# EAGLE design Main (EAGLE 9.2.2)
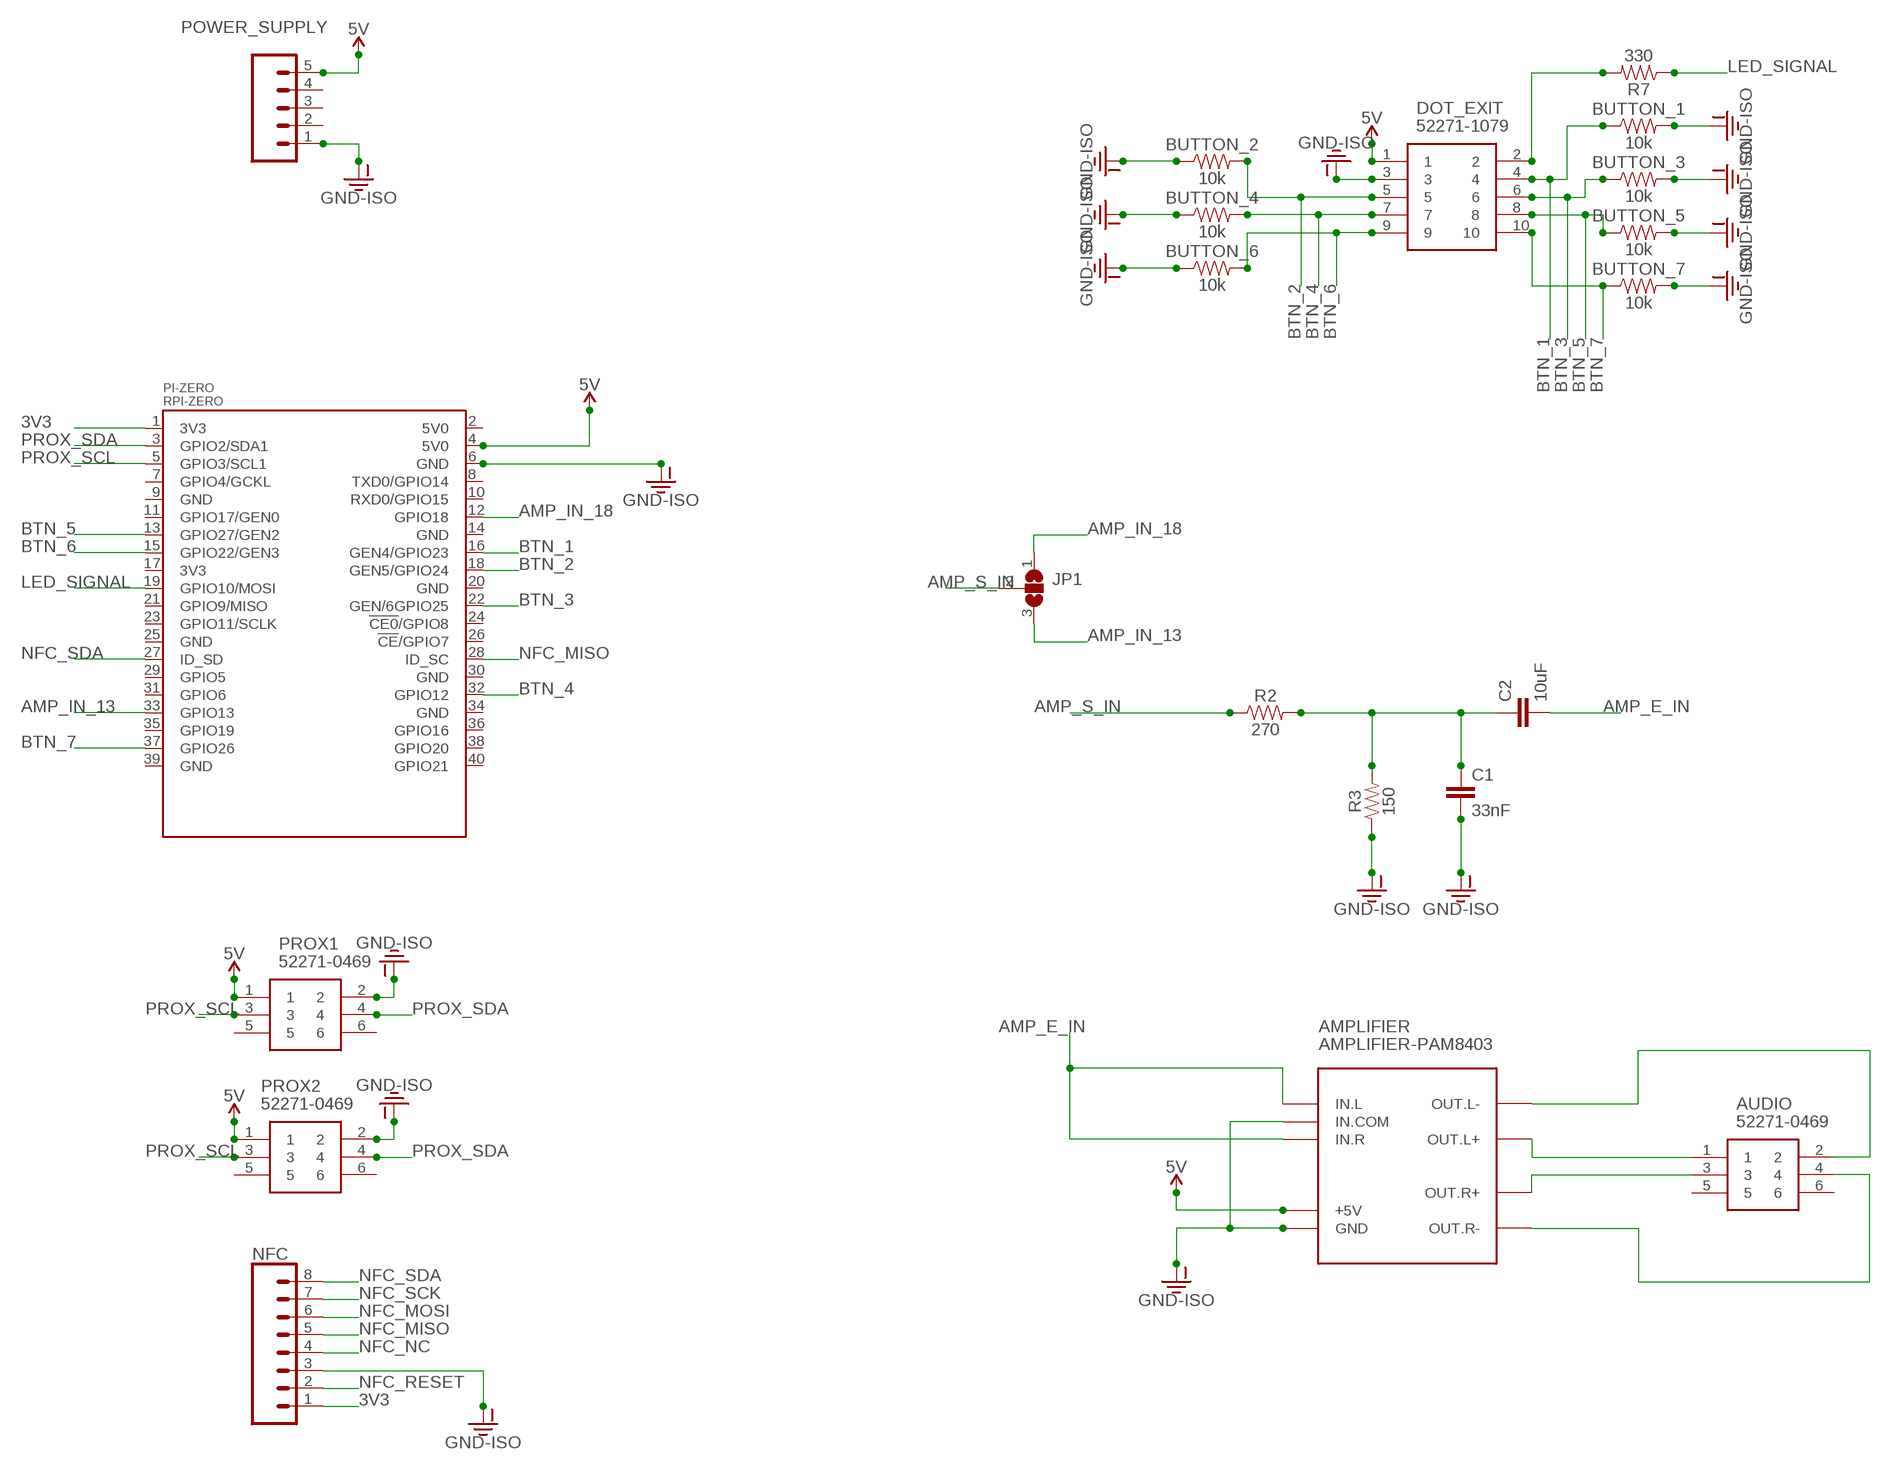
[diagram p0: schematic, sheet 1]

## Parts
AMPLIFIER  AMPLIFIER-PAM8403  [AMPLIFIER-PAM8403]
AUDIO  52271-0469  [MOLEX_52271-0469]
BUTTON_1  10k  1KOHM-HORIZ-1/4W-1%  [AXIAL-0.3]
BUTTON_2  10k  1KOHM-HORIZ-1/4W-1%  [AXIAL-0.3]
BUTTON_3  10k  1KOHM-HORIZ-1/4W-1%  [AXIAL-0.3]
BUTTON_4  10k  1KOHM-HORIZ-1/4W-1%  [AXIAL-0.3]
BUTTON_5  10k  1KOHM-HORIZ-1/4W-1%  [AXIAL-0.3]
BUTTON_6  10k  1KOHM-HORIZ-1/4W-1%  [AXIAL-0.3]
BUTTON_7  10k  1KOHM-HORIZ-1/4W-1%  [AXIAL-0.3]
C1  33nF  10NF-PTH-10MM-10000V-1-%  [CAP-PTH-10MM]
C2  10uF  10NF-PTH-10MM-10000V-1-%  [CAP-PTH-10MM]
DOT_EXIT  52271-1079  [52271-1079]
JP1  SJ2W  [SJ_2]
NFC  CONN_08"  [1X08]
PI-ZERO  RPI-ZERO  [RASPBERRYPI_BASTELSTUBE_V13_RASPI_BOARD_B+_FULL]
POWER_SUPPLY  CONN_05  [1X05]
PROX1  52271-0469  [MOLEX_52271-0469]
PROX2  52271-0469  [MOLEX_52271-0469]
R2  270  330OHM-HORIZ-1/10W-5%  [AXIAL-0.3]
R3  150  330OHM-HORIZ-1/10W-5%  [AXIAL-0.3]
R7  330  330OHM-HORIZ-1/10W-5%  [AXIAL-0.3]

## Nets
3V3: NFC.1 PI-ZERO.1(3V3)
5V [power]: AMPLIFIER.+5V DOT_EXIT.1 PI-ZERO.4(5V0) POWER_SUPPLY.5 PROX1.1 PROX2.1
AMP_E_IN: AMPLIFIER.IN.L AMPLIFIER.IN.R C2.2
AMP_IN_13: JP1.3 PI-ZERO.33(GPIO13)
AMP_IN_18: JP1.1 PI-ZERO.12(GPIO18)
AMP_S_IN: JP1.2 R2.P$1
BTN_1: BUTTON_1.P$1 DOT_EXIT.4 PI-ZERO.16(GEN4/GPIO23)
BTN_2: BUTTON_2.P$2 DOT_EXIT.5 PI-ZERO.18(GEN5/GPIO24)
BTN_3: BUTTON_3.P$1 DOT_EXIT.6 PI-ZERO.22(GEN/6GPIO25)
BTN_4: BUTTON_4.P$2 DOT_EXIT.7 PI-ZERO.32(GPIO12)
BTN_5: BUTTON_5.P$1 DOT_EXIT.8 PI-ZERO.13(GPIO27/GEN2)
BTN_6: BUTTON_6.P$2 DOT_EXIT.9 PI-ZERO.15(GPIO22/GEN3)
BTN_7: BUTTON_7.P$1 DOT_EXIT.10 PI-ZERO.37(GPIO26)
GND-ISO [power]: AMPLIFIER.GND AMPLIFIER.IN.COM BUTTON_1.P$2 BUTTON_2.P$1 BUTTON_3.P$2 BUTTON_4.P$1 BUTTON_5.P$2 BUTTON_6.P$1 BUTTON_7.P$2 C1.2 DOT_EXIT.3 NFC.3 PI-ZERO.6(GND) POWER_SUPPLY.1 PROX1.2 PROX2.2 R3.P$1
LED_SIGNAL: PI-ZERO.19(GPIO10/MOSI) R7.P$1
N$1: DOT_EXIT.2 R7.P$2
N$2: AMPLIFIER.OUT.L- AUDIO.2
N$3: AMPLIFIER.OUT.L+ AUDIO.1
N$4: C1.1 C2.1 R2.P$2 R3.P$2
N$5: AMPLIFIER.OUT.R+ AUDIO.3
N$6: AMPLIFIER.OUT.R- AUDIO.4
NFC_MISO: NFC.5 PI-ZERO.28(ID_SC)
NFC_MOSI: NFC.6
NFC_NC: NFC.4
NFC_RESET: NFC.2
NFC_SCK: NFC.7
NFC_SDA: NFC.8 PI-ZERO.27(ID_SD)
PROX_SCL: PI-ZERO.5(GPIO3/SCL1) PROX1.3 PROX2.3
PROX_SDA: PI-ZERO.3(GPIO2/SDA1) PROX1.4 PROX2.4
Unconnected: AUDIO.5 AUDIO.6 PI-ZERO.2(5V0) PI-ZERO.7(GPIO4/GCKL) PI-ZERO.8(TXD0/GPIO14) PI-ZERO.9(GND) PI-ZERO.10(RXD0/GPIO15) PI-ZERO.11(GPIO17/GEN0) PI-ZERO.14(GND) PI-ZERO.17(3V3) PI-ZERO.20(GND) PI-ZERO.21(GPIO9/MISO) PI-ZERO.23(GPIO11/SCLK) PI-ZERO.24(!CE0!/GPIO8) PI-ZERO.25(GND) PI-ZERO.26(!CE!/GPIO7) PI-ZERO.29(GPIO5) PI-ZERO.30(GND) PI-ZERO.31(GPIO6) PI-ZERO.34(GND) PI-ZERO.35(GPIO19) PI-ZERO.36(GPIO16) PI-ZERO.38(GPIO20) PI-ZERO.39(GND) PI-ZERO.40(GPIO21) POWER_SUPPLY.2 POWER_SUPPLY.3 POWER_SUPPLY.4 PROX1.5 PROX1.6 PROX2.5 PROX2.6

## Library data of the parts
AMPLIFIER = diy-modules:AMPLIFIER-PAM8403: Stereo Class-D 3W Audio Amplifier based on PAM8403 chip More details available here: http://artofcircuits.com/product/pam8403-5v-two-channel-stereo-mini-class-d-3w3w-audio-amplifier Click here to find device on ebay.com
AUDIO PROX1 PROX2 = 52271-0469:52271-0469: CONNECTOR, FPC, 1.0MM, 4 WAY Source: Datasheet; ALLIED_NUMBER: 70374312; DESCRIPTION: CONNECTOR, FPC, 1.0MM, 4 WAY; HEIGHT: mm; MANUFACTURER_NAME: Molex; MANUFACTURER_PART_NUMBER: 52271-0469; RS_PART_NUMBER: 1707199
BUTTON_1-BUTTON_7 = SparkFun-Resistors:1KOHM: 1kΩ resistor; PROD_ID: RES-12182; VALUE: 1k
C1 C2 = SparkFun-Capacitors:10NF: 0.01uF/10nF/10,000pF ceramic capacitors; PROD_ID: CAP-09321; VALUE: 10nF
DOT_EXIT = 52271-1079:52271-1079: 1.0MM FPC R/A CONN 10 W Molex FFC/FPC SMT Series 1mm Pitch 10 Way Right Angle SMT Female FPC Connector, ZIF Bottom Contact Source: Datasheet; ALLIED_NUMBER: 70373119; DESCRIPTION: 1.0MM FPC R/A CONN 10 W Molex FFC/FPC SMT Series 1mm Pitch 10 Way Right Angle SMT Female FPC Connector, ZIF Bottom Contact; HEIGHT: mm; MANUFACTURER_NAME: Molex; MANUFACTURER_PART_NUMBER: 52271-1079; RS_PART_NUMBER: 5144329P
JP1 = jumper:SJ2W: SMD solder JUMPER
NFC = SparkFun-Connectors:CONN_08: Multi connection point. Often used as Generic Header-pin footprint for 0.1 inch spaced/style header connections On any of the 0.1 inch spaced packages, you can populate with these: Break Away Headers - Straight (PRT-00116) Break Away Male Headers - Right Angle (PRT-00553) Female Headers (PRT-00115)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; PROD_ID: CONN-08438
PI-ZERO = RPI-Zero-Footprint:RPI-ZERO
POWER_SUPPLY = SparkFun-Connectors:CONN_05: Multi connection point. Often used as Generic Header-pin footprint for 0.1 inch spaced/style header connections On any of the 0.1 inch spaced packages, you can populate with these: Break Away Headers - Straight (PRT-00116) Break Away Male Headers - Right Angle (PRT-00553) Female Headers (PRT-00115)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
R2 R3 = SparkFun-Resistors:330OHM: 330Ω resistor; PROD_ID: RES-8371; VALUE: 330
R7 = SparkFun-Resistors:330OHM: 330Ω resistor; PROD_ID: RES-8371

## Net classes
0 default: width 0.254 mm, drill 0.508 mm, clearance 0.254 mm
1 power: width 0.508 mm, drill 0.635 mm, clearance 0.381 mm

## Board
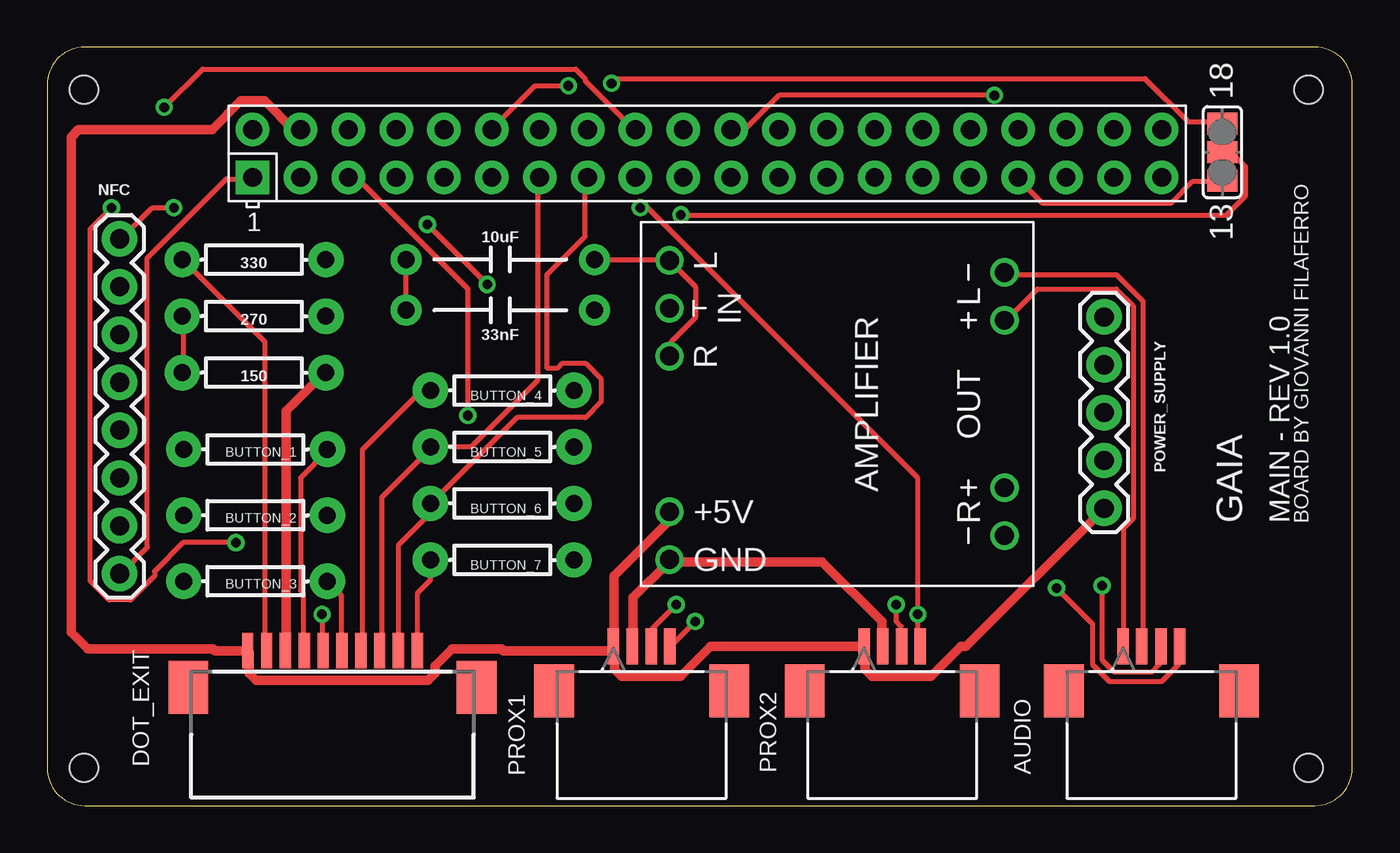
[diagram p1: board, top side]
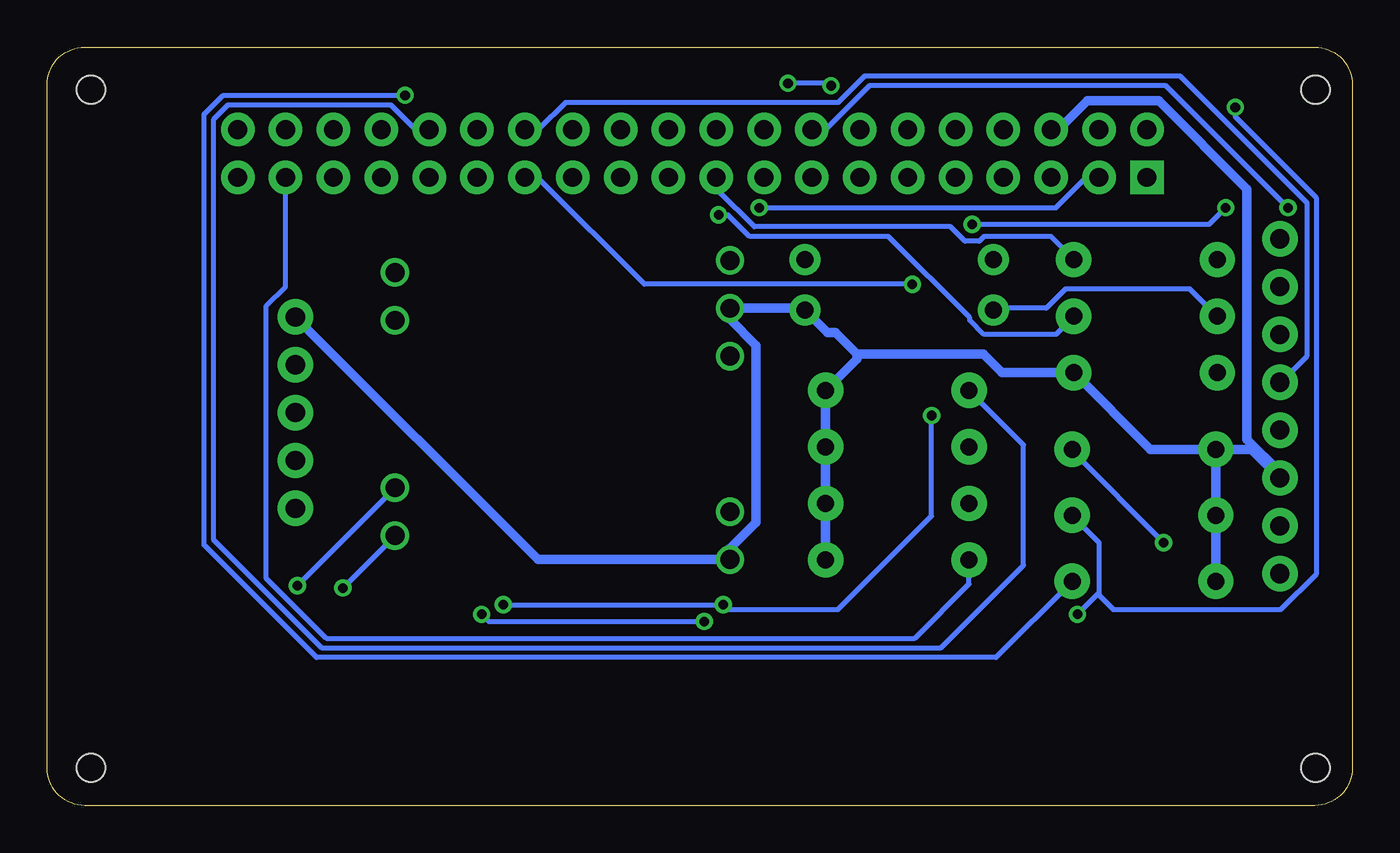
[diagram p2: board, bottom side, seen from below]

Size 69.29 x 40.27 mm. Coordinates in mm from the lower left corner, seen from the top.
Outline: 0,38.27 0,2 arc90 2,0 67.29,0 arc90 69.29,2 69.29,38.27 arc90 67.29,40.27 2,40.27 arc90 0,38.27
Copper layers (1*16): Top 0.035mm / dielectric 1.5mm / Bottom 0.035mm
Design rules "default": minimum track width 6mil, minimum drill 0.35mm, track to track 6mil, track to pad 6mil, pad to pad 6mil, via to via 6mil, smd to smd 6mil, copper to edge 40mil, drill to drill 6mil, minimum pad ring 10mil, minimum via ring 8mil, stop-mask expansion 4mil, vias tented up to drill 0mil, thermal gap 10mil
Holes 1.5 mm at 1.96,38 66.96,38 66.96,2 1.96,2

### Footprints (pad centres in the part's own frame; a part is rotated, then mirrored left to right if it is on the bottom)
AMPLIFIER-PAM8403 = drill 1: +5V 5.715,-8.89; GND 8.255,-8.89; IN.COM -5.08,-8.89; IN.L -7.62,-8.89; IN.R -2.54,-8.89; OUT.L+ -4.445,8.89; OUT.L- -6.985,8.89; OUT.R+ 4.445,8.89; OUT.R- 6.985,8.89
MOLEX_52271-0469 = smd 0.61 x 1.905: 1 1.499,4.699; 2 0.508,4.699; 3 -0.508,4.699; 4 -1.499,4.699 | smd 2.108 x 2.794: 5 -4.648,7.061; 6 4.648,7.061
AXIAL-0.3 = drill 0.9 pad 1.88: P$1 -3.81,0; P$2 3.81,0
CAP-PTH-10MM = drill 0.9 pad 1.651: 1 -5,0; 2 5,0
52271-1079 = smd 0.6 x 1.9: 1 -4.5,1.1; 2 -3.5,1.1; 3 -2.5,1.1; 4 -1.5,1.1; 5 -0.5,1.1; 6 0.5,1.1; 7 1.5,1.1; 8 2.5,1.1; 9 3.5,1.1; 10 4.5,1.1 | smd 2.1 x 2.8: 11 7.65,-0.85; 12 -7.65,-0.85
SJ_2 = smd 1.168 x 1.6: 1 -1.524,0; 2 0,0; 3 1.524,0
1X08 = drill 1.016 pad 1.88: 1 0,0; 2 2.54,0; 3 5.08,0; 4 7.62,0; 5 10.16,0; 6 12.7,0; 7 15.24,0; 8 17.78,0
RASPBERRYPI_BASTELSTUBE_V13_RASPI_BOARD_B+_FULL = drill 1 pad 1.778 square: 1 8.37,25.23 | drill 1 pad 1.778: 2 8.37,27.77; 3 10.91,25.23; 4 10.91,27.77; 5 13.45,25.23; 6 13.45,27.77; 7 15.99,25.23; 8 15.99,27.77; 9 18.53,25.23; 10 18.53,27.77; 11 21.07,25.23; 12 21.07,27.77; 13 23.61,25.23; 14 23.61,27.77; 15 26.15,25.23; 16 26.15,27.77; 17 28.69,25.23; 18 28.69,27.77; 19 31.23,25.23; 20 31.23,27.77; 21 33.77,25.23; 22 33.77,27.77; 23 36.31,25.23; 24 36.31,27.77; 25 38.85,25.23; 26 38.85,27.77; 27 41.39,25.23; 28 41.39,27.77; 29 43.93,25.23; 30 43.93,27.77; 31 46.47,25.23; 32 46.47,27.77; 33 49.01,25.23; 34 49.01,27.77; 35 51.55,25.23; 36 51.55,27.77; 37 54.09,25.23; 38 54.09,27.77; 39 56.63,25.23; 40 56.63,27.77
1X05 = drill 1.016 pad 1.88: 1 0,0; 2 2.54,0; 3 5.08,0; 4 7.62,0; 5 10.16,0

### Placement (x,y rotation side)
AMPLIFIER  41.93,21.32 270 top
AUDIO  58.62,13.15 180 top
BUTTON_1  11.06,18.91 180 top
BUTTON_2  11.06,15.41 0 top
BUTTON_3  11.06,11.91 180 top
BUTTON_4  24.16,22.04 180 top
BUTTON_5  24.16,19.04 0 top
BUTTON_6  24.16,16.04 180 top
BUTTON_7  24.16,13.04 0 top
C1  24.05,26.3 0 top
C2  24.05,28.99 0 top
DOT_EXIT  15.15,7.12 0 top
JP1  62.38,34.69 270 top
NFC  3.85,12.31 90 top
PI-ZERO  2.54,8.12 0 top
POWER_SUPPLY  56.11,25.94 270 top
PROX1  31.56,13.15 180 top
PROX2  44.86,13.15 180 top
R2  10.98,25.98 180 top
R3  10.98,22.98 180 top
R7  10.98,28.98 180 top

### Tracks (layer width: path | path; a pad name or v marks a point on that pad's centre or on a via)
3V3
  Top 0.254: PI-ZERO.1 10.79,33.27 9.52,33.27 5.33,29.07 5.33,13.71 3.93,12.31 NFC.1
5V
  Top 0.508: POWER_SUPPLY.5 48.78,8.45 48.51,8.45 46.93,6.86 43.78,6.86 43.41,7.23 43.41,8.4 PROX2.1 35.21,8.45 33.63,6.86 30.48,6.86 30.11,7.23 30.11,8.4 PROX1.1 | PROX1.1 29.83,8.22 24.2,8.22 24.11,8.3 21.49,8.3 20.59,7.4 20.59,7.01 20.21,6.63 11.09,6.63 10.71,7.01 10.71,8.16 DOT_EXIT.1 8.9,8.22 8.81,8.3 2.16,8.3 1.27,9.19 1.27,35.5 1.66,35.89 8.75,35.89 10.28,37.41 11.54,37.41 13.07,35.89 PI-ZERO.4 | AMPLIFIER.+5V 33.01,15.49 33.01,15.11 30.09,12.18 30.09,8.63 PROX1.1
AMP_E_IN
  Top 0.254: AMPLIFIER.IN.R 33.14,23.87 33.14,24.63 34.41,25.9 34.41,27.55 33.14,28.82 AMPLIFIER.IN.L 33.01,28.95 29.07,28.95 C2.2
AMP_IN_13
  Top 0.254: JP1.3 62.35,33.14 60.83,33.14 59.68,32 52.82,32 51.55,33.27 PI-ZERO.33
AMP_IN_18  (via drill 0.51)
  Top 0.254: v29.96,38.35 30.22,38.6 58.29,38.6 60.57,36.31 62.35,36.31 JP1.1 | v27.68,38.22 25.9,38.22 23.61,35.93 PI-ZERO.12
  Bottom 0.254: v29.96,38.35 27.8,38.35 v27.68,38.22
AMP_S_IN  (via drill 0.51)
  Top 0.254: v33.65,31.36 62.6,31.36 63.62,32.38 63.62,33.9 62.86,34.66 62.48,34.66 JP1.2
  Bottom 0.254: v33.65,31.36 33.14,31.36 32,30.22 24.63,30.22 20.31,25.9 20.31,25.77 19.55,25.01 15.74,25.01 14.85,25.9 R2.P$1
BTN_1  (via drill 0.51)
  Top 0.254: DOT_EXIT.4 13.58,8.25 13.58,11.29 13.45,11.42 13.45,17.39 14.85,18.79 BUTTON_1.P$1 | v3.42,31.74 2.28,30.6 2.28,11.93 3.29,10.91 4.44,10.91 5.71,12.18 5.71,12.44 7.23,13.96 v10.02,13.96
  Bottom 0.254: v3.42,31.74 9.9,38.22 25.65,38.22 27.93,35.93 28.57,35.93 PI-ZERO.16 | v10.02,13.96 14.85,18.79 BUTTON_1.P$1
BTN_2  (via drill 0.51)
  Top 0.254: v14.6,10.15 14.6,8.25 DOT_EXIT.5 | v6.22,37.08 8.25,39.11 28.06,39.11 28.57,38.6 28.57,38.47 31.11,35.93 PI-ZERO.18
  Bottom 0.254: 13.52,11.23 13.45,11.29 13.45,13.96 14.85,15.36 BUTTON_2.P$2 | 13.52,11.23 v14.6,10.15 | v6.22,37.08 6.22,36.57 1.9,32.25 1.9,12.31 3.8,10.41 12.69,10.41 13.52,11.23
BTN_3  (via drill 0.51)
  Top 0.254: DOT_EXIT.6 15.61,8.25 15.61,11.17 14.98,11.8 BUTTON_3.P$1 | v50.28,37.71 38.85,37.71 37.08,35.93 36.31,35.93 PI-ZERO.22
  Bottom 0.254: v50.28,37.71 59.94,37.71 60.95,36.7 60.95,13.84 54.98,7.87 18.91,7.87 14.98,11.8 BUTTON_3.P$1
BTN_4
  Top 0.254: DOT_EXIT.7 16.76,8.25 16.76,18.91 19.88,22.04 BUTTON_4.P$2
  Bottom 0.254: PI-ZERO.32 49.01,35.93 49.78,35.93 51.05,37.2 59.68,37.2 60.44,36.44 60.44,14.09 54.73,8.37 21.84,8.37 17.46,12.75 17.46,19.15 BUTTON_4.P$2
BTN_5
  Top 0.254: DOT_EXIT.8 17.77,8.25 17.77,16.38 20.35,18.95 BUTTON_5.P$1 22.5,19.04 26.03,22.57 26.03,33.27 PI-ZERO.13
BTN_6
  Top 0.254: DOT_EXIT.9 18.66,8.25 18.66,13.84 20.35,15.52 20.35,16 | PI-ZERO.15 28.57,33.27 28.57,30.22 26.54,28.19 26.54,23.23 27.12,23.23 27.37,23.49 28.57,23.49 29.42,22.64 29.42,21.44 28.57,20.59 24.94,20.59 20.35,16 | 20.35,16 BUTTON_6.P$2
BTN_7
  Top 0.254: DOT_EXIT.10 19.68,8.25 19.68,11.29 20.35,11.97 BUTTON_7.P$1
  Bottom 0.254: PI-ZERO.37 56.63,33.27 56.63,27.55 57.65,26.54 57.65,12.06 54.48,8.88 23.23,8.88 20.35,11.77 BUTTON_7.P$1
GND-ISO
  Top 0.508: 12.59,8.29 DOT_EXIT.3 12.69,8.5 12.69,20.95 14.72,22.98 R3.P$1 | PROX1.2 31.11,8.5 31.11,11.04 33.01,12.95 AMPLIFIER.GND 33.27,12.95 41.14,12.95 44.31,9.77 44.31,8.5 PROX2.2
  Bottom 0.508: POWER_SUPPLY.1 43.23,13.06 AMPLIFIER.GND 33.04,13.64 31.65,15.03 31.65,24.43 33.04,25.82 AMPLIFIER.IN.COM 29.15,26.4 C1.2 27.87,25.12 27.43,25.12 26.3,23.98 | PI-ZERO.6 15.61,35.89 14.08,37.41 10.28,37.41 5.59,32.73 5.59,19.45 3.85,17.7 NFC.3 5.37,18.91 BUTTON_1.P$2 | BUTTON_1.P$2 BUTTON_2.P$1 BUTTON_3.P$2 | BUTTON_1.P$2 10.71,18.91 R3.P$1 18.6,22.98 19.6,23.98 26.3,23.98 | 26.3,23.98 26.3,23.71 BUTTON_4.P$1 BUTTON_5.P$2 BUTTON_6.P$1 BUTTON_7.P$2
LED_SIGNAL
  Bottom 0.254: PI-ZERO.19 33.65,33.27 33.65,32.63 31.74,30.73 21.33,30.73 20.57,29.96 19.8,29.96 19.55,30.22 15.99,30.22 14.85,29.07 R7.P$1
N$1
  Top 0.254: DOT_EXIT.2 11.55,8.25 11.55,24.63 7.23,28.95 R7.P$2
N$2
  Top 0.254: AUDIO.2 58.16,8.5 58.16,26.79 56.76,28.19 50.92,28.19 AMPLIFIER.OUT.L-
N$3
  Top 0.254: AUDIO.1 57.14,8.5 57.14,14.72 57.65,15.23 57.65,26.54 56.76,27.42 52.57,27.42 50.92,25.77 AMPLIFIER.OUT.L+
N$4
  Top 0.254: C1.1 19.04,26.41 19.04,28.95 C2.1 | R3.P$2 7.23,23.11 7.23,25.9 R2.P$2
  Bottom 0.254: C1.1 19.04,26.41 16.25,26.41 15.23,27.42 8.63,27.42 7.23,26.03 R2.P$2
N$5  (via drill 0.51)
  Top 0.254: v56,11.68 56,7.74 56.63,7.1 58.67,7.1 59.05,7.49 59.05,8.37 AUDIO.3
  Bottom 0.254: v56,11.68 50.92,16.76 AMPLIFIER.OUT.R+
N$6  (via drill 0.51)
  Top 0.254: v53.59,11.55 55.49,9.64 55.49,7.49 56.38,6.6 59.17,6.6 60.06,7.49 60.06,8.37 AUDIO.4
  Bottom 0.254: v53.59,11.55 50.92,14.22 AMPLIFIER.OUT.R-
NFC_MISO
  Bottom 0.254: PI-ZERO.28 43.81,35.93 43.17,35.93 41.77,37.33 27.3,37.33 25.9,38.73 9.14,38.73 2.41,32 2.41,23.87 3.8,22.47 NFC.5
NFC_SDA  (via drill 0.51)
  Top 0.254: v20.19,30.85 v23.36,27.68 | v6.72,31.74 5.58,31.74 3.93,30.09 NFC.8
  Bottom 0.254: v23.36,27.68 37.58,27.68 43.17,33.27 43.81,33.27 PI-ZERO.27 | v20.19,30.85 7.61,30.85 v6.72,31.74
PROX_SCL  (via drill 0.51)
  Top 0.254: v33.39,10.66 32.12,9.39 32.12,8.5 PROX1.3 | v45.08,10.66 45.08,9.77 45.33,9.52 45.33,8.5 PROX2.3 | v22.34,20.71 22.34,27.43 16.5,33.27 15.99,33.27 PI-ZERO.5
  Bottom 0.254: v45.08,10.66 v33.39,10.66 33.14,10.41 27.3,10.41 22.34,15.37 v22.34,20.71
PROX_SDA  (via drill 0.51)
  Top 0.254: v34.41,9.77 33.14,8.5 PROX1.4 | PROX2.4 46.35,8.5 46.22,8.63 v46.22,10.15 46.22,17.39 31.87,31.74 v31.49,31.74
  Bottom 0.254: v34.41,9.77 45.84,9.77 v46.22,10.15 | v31.49,31.74 15.74,31.74 14.22,33.27 13.45,33.27 PI-ZERO.3

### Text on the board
tNames: 18 | 13 | BUTTON_4 | BUTTON_1 | BUTTON_5 | BUTTON_6 | BUTTON_2 | GAIA | MAIN - REV 1.0 | BOARD BY GIOVANNI FILAFERRO | BUTTON_7 | BUTTON_3

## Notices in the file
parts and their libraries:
SparkFun-Connectors: Licensing: Creative Commons ShareAlike 4.0 International - https://creativecommons.org/licenses/by-sa/4.0
diy-modules: Released under the Creative Commons Attribution 4.0 International License: http://creativecommons.org/licenses/by/4.0
